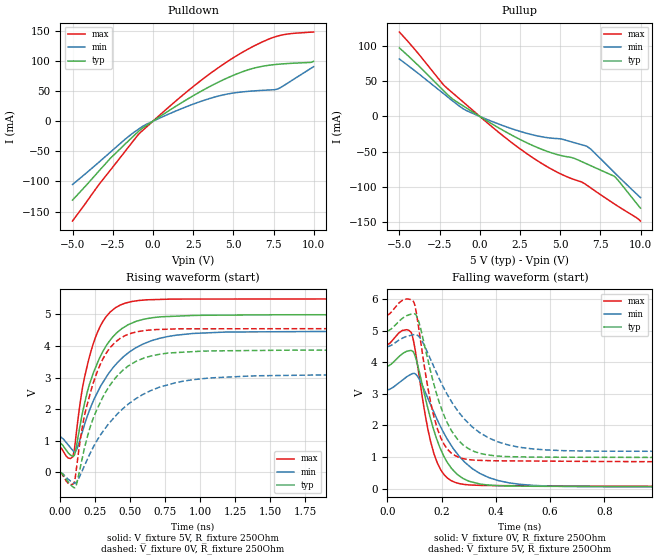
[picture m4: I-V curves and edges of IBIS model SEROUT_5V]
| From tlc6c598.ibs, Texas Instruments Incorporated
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|   Model SEROUT_5V
[Model]   SEROUT_5V
Model_type   Output
Polarity   Inverting
Vmeas = 2.5
Vref = 5
Cref = 0pF
Rref = 250
|   typ   min   max
|   (nom PVT)   (fast PVT)   (slow PVT)
C_comp   1.348p   1.226p   1.507p
|C_comp (Hi state)   1.477p   1.432p   1.548p
|C_comp (Low state)   1.348p   1.226p   1.507p
[Voltage Range]   5   4.5   5.5
[Temperature Range]   27   150   -40
[Pullup Reference]   5   4.5   5.5
[Pulldown Reference]   -0   -0   -0
[Power Clamp Reference]   5   4.5   5.5
[GND Clamp Reference]   -0   -0   -0
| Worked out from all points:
|   slope of the pulldown table from 0 to 0.75 V, typ, clamps not added: 56.6 ohm
|   slope of the pullup table from 0 to 0.75 V, typ, clamps not added: 71.1 ohm
|   falling waveform, V_fixture 0V, R_fixture 250Ohm: 20-80 % time 89.9ps typ, 144ps min, 63.3ps max; typ from 3.88 V to 0.028 V
|   rising waveform, V_fixture 5V, R_fixture 250Ohm: 20-80 % time 203ps typ, 300ps min, 150ps max; typ from 0.926 V to 4.99 V
|   rising waveform, V_fixture 0V, R_fixture 250Ohm: 20-80 % time 243ps typ, 383ps min, 172ps max; typ from 0 V to 3.87 V
|   falling waveform, V_fixture 5V, R_fixture 250Ohm: 20-80 % time 95.9ps typ, 160ps min, 66.3ps max; typ from 5 V to 0.95 V
[Pulldown]
|   Voltage   I(typ)   I(min)   I(max)
-5V       -130.9mA   -105.1mA   -165.6mA
-3.335V   -82.03mA   -67.47mA   -104.3mA
-2.645V   -61.54mA   -51.33mA   -81.14mA
-920mV    -17.51mA   -13.67mA   -22.59mA
415mV     7.388mA    5.1mA      9.966mA
2.785V    46.55mA    31.05mA    63.38mA
3.985V    63.65mA    41.11mA    87.23mA
5.035V    76.49mA    46.9mA     105.8mA
6.805V    91.13mA    51.19mA    131.6mA
7.765V    94.44mA    53.5mA     141.3mA
8.725V    96.21mA    69.12mA    145.7mA
9.985V    99.32mA    90.4mA     147.9mA
[Pullup]
|   Voltage   I(typ)   I(min)   I(max)
-5V       97.62mA    81.79mA    120.2mA
-3.92V    74.7mA     62.91mA    92.16mA
-2.27V    37.06mA    32.76mA    45.32mA
-1.655V   24.16mA    21.46mA    32.77mA
-1.04V    15.09mA    11mA       20.67mA
1.675V    -22.79mA   -15.04mA   -31.83mA
4.195V    -49.84mA   -30.25mA   -71.74mA
5.08V     -55.87mA   -32.23mA   -82.47mA
5.875V    -59.77mA   -37.42mA   -90.01mA
6.655V    -67.71mA   -42.56mA   -97.97mA
8.395V    -85.9mA    -80.59mA   -125.1mA
9.985V    -130.7mA   -115.6mA   -149mA
[Ramp]
R_load = 250
|   typ   min   max
dV/dt_r   2.43833/2.034e-10   2.01527/3.0013e-10   2.81997/1.50128e-10
dV/dt_f   2.31258/8.99827e-11   1.85919/1.43672e-10   2.72295/6.33735e-11
[Falling Waveform]
V_fixture = 0V
V_fixture_min = 0V
V_fixture_max = 0V
R_fixture = 250Ohm
C_fixture = 0F
|   Time   V(typ)   V(min)   V(max)
0s        3.882V     3.13V      4.561V
87.56ps   4.379V     3.624V     4.957V
105.8ps   4.109V     3.615V     4.223V
141.2ps   2.834V     3.026V     2.255V
172ps     1.837V     2.413V     1.1V
209.6ps   1.007V     1.742V     435.6mV
265.2ps   402.9mV    1.021V     157.4mV
374.1ps   111.2mV    347.6mV    95.95mV
587.2ps   71.36mV    81.91mV    82.91mV
2.9ns     27.91mV    30.87mV    22.78mV
[Rising Waveform]
V_fixture = 5V
V_fixture_min = 4.5V
V_fixture_max = 5.5V
R_fixture = 250Ohm
C_fixture = 0F
|   Time   V(typ)   V(min)   V(max)
0s        925.5mV    1.125V     789.6mV
71.72ps   549.4mV    783.1mV    439.7mV
98.74ps   538.4mV    647.8mV    708.1mV
159.4ps   1.926V     1.326V     2.727V
249.9ps   3.31V      2.405V     4.268V
355.1ps   4.181V     3.194V     5.072V
465.6ps   4.623V     3.715V     5.359V
647.2ps   4.887V     4.162V     5.463V
947.2ps   4.965V     4.395V     5.483V
2.9ns     4.989V     4.484V     5.49V
[Rising Waveform]
V_fixture = 0V
V_fixture_min = 0V
V_fixture_max = 0V
R_fixture = 250Ohm
C_fixture = 0F
|   Time   V(typ)   V(min)   V(max)
0s        706.1pV    96.86nV    525.3pV
71.72ps   -387.8mV   -271.4mV   -381.9mV
105.8ps   -479.2mV   -336.5mV   -160.5mV
172ps     774.1mV    215.3mV    1.803V
265.2ps   2.035V     1.04V      3.214V
355.1ps   2.765V     1.593V     3.949V
511ps     3.437V     2.245V     4.409V
707.2ps   3.737V     2.696V     4.522V
1.067ns   3.842V     2.988V     4.543V
2.9ns     3.871V     3.104V     4.55V
[Falling Waveform]
|Gnd
V_fixture = 5V
V_fixture_min = 4.5V
V_fixture_max = 5.5V
R_fixture = 250Ohm
C_fixture = 0F
|   Time   V(typ)   V(min)   V(max)
0s        5V         4.5V       5.5V
97.58ps   5.539V     4.881V     5.911V
115.7ps   5.297V     4.825V     5.082V
149.4ps   4.08V      4.29V      3.195V
184.5ps   2.921V     3.609V     1.893V
222.1ps   2.066V     2.965V     1.243V
283.8ps   1.357V     2.206V     940.8mV
407.5ps   1.031V     1.48V      880.4mV
587.2ps   995.6mV    1.224V     870.1mV
2.9ns     949.5mV    1.152V     808.6mV
